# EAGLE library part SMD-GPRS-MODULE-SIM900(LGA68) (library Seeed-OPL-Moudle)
317040000
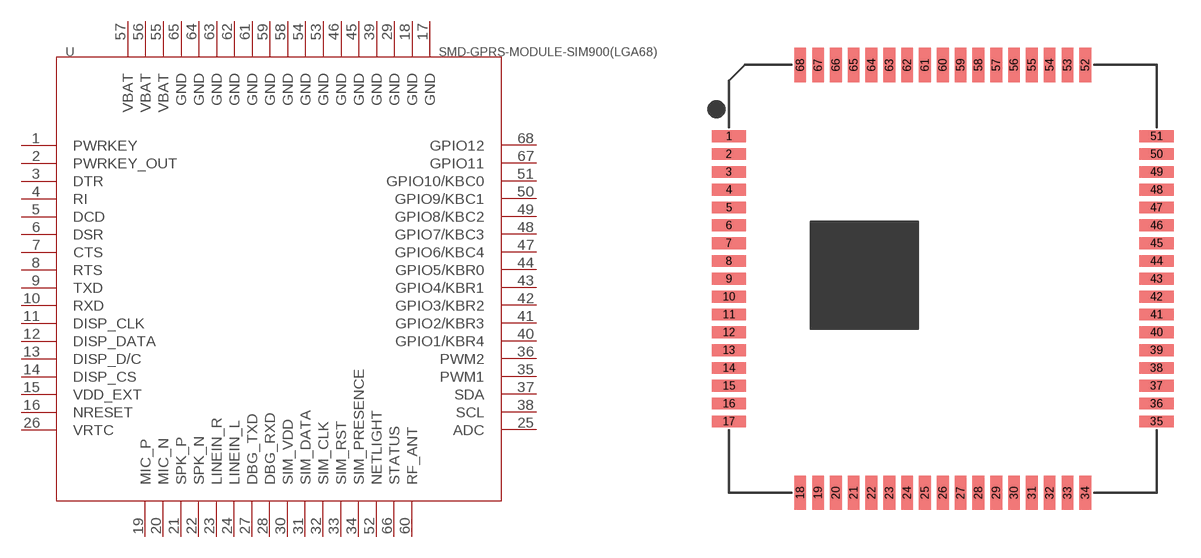
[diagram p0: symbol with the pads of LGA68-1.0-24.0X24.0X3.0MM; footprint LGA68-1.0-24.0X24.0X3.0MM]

Designator prefix U

## SMD-GPRS-MODULE-SIM900(LGA68) (MPN: SIM900; VALUE: SIM900)  [LGA68-1.0-24.0X24.0X3.0MM]
1  PWRKEY  in
2  PWRKEY_OUT  out
3  DTR  in
4  RI  out
5  DCD  out
6  DSR  out
7  CTS  out
8  RTS  in
9  TXD  out
10  RXD  in
11  DISP_CLK  out
12  DISP_DATA
13  DISP_D/C  out
14  DISP_CS  out
15  VDD_EXT  out
16  NRESET  in
17  GND  pwr
18  GND  pwr
19  MIC_P  in
20  MIC_N  in
21  SPK_P  out
22  SPK_N  out
23  LINEIN_R  in
24  LINEIN_L  in
25  ADC  in
26  VRTC
27  DBG_TXD  out
28  DBG_RXD  in
29  GND  pwr
30  SIM_VDD  out
31  SIM_DATA
32  SIM_CLK  out
33  SIM_RST  out
34  SIM_PRESENCE  in
35  PWM1  out
36  PWM2  out
37  SDA
38  SCL  out
39  GND  pwr
40  GPIO1/KBR4  out
41  GPIO2/KBR3  out
42  GPIO3/KBR2  out
43  GPIO4/KBR1  out
44  GPIO5/KBR0  out
45  GND  pwr
46  GND  pwr
47  GPIO6/KBC4  in
48  GPIO7/KBC3
49  GPIO8/KBC2  in
50  GPIO9/KBC1  in
51  GPIO10/KBC0
52  NETLIGHT  out
53  GND  pwr
54  GND  pwr
55  VBAT  pwr
56  VBAT  pwr
57  VBAT  pwr
58  GND  pwr
59  GND  pwr
60  RF_ANT
61  GND  pwr
62  GND  pwr
63  GND  pwr
64  GND  pwr
65  GND  pwr
66  STATUS  out
67  GPIO11
68  GPIO12

## Footprint LGA68-1.0-24.0X24.0X3.0MM (pad centres in mm)
smd 1.93 x 0.66: 1 -12,8; 2 -12,7; 3 -12,6; 4 -12,5; 5 -12,4; 6 -12,3; 7 -12,2; 8 -12,1; 9 -12,0; 10 -12,-1; 11 -12,-2; 12 -12,-3; 13 -12,-4; 14 -12,-5; 15 -12,-6; 16 -12,-7; 17 -12,-8; 35 12,-8; 36 12,-7; 37 12,-6; 38 12,-5; 39 12,-4; 40 12,-3; 41 12,-2; 42 12,-1; 43 12,0; 44 12,1; 45 12,2; 46 12,3; 47 12,4; 48 12,5; 49 12,6; 50 12,7; 51 12,8
smd 0.66 x 1.93: 18 -8,-12; 19 -7,-12; 20 -6,-12; 21 -5,-12; 22 -4,-12; 23 -3,-12; 24 -2,-12; 25 -1,-12; 26 0,-12; 27 1,-12; 28 2,-12; 29 3,-12; 30 4,-12; 31 5,-12; 32 6,-12; 33 7,-12; 34 8,-12; 52 8,12; 53 7,12; 54 6,12; 55 5,12; 56 4,12; 57 3,12; 58 2,12; 59 1,12; 60 0,12; 61 -1,12; 62 -2,12; 63 -3,12; 64 -4,12; 65 -5,12; 66 -6,12; 67 -7,12; 68 -8,12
